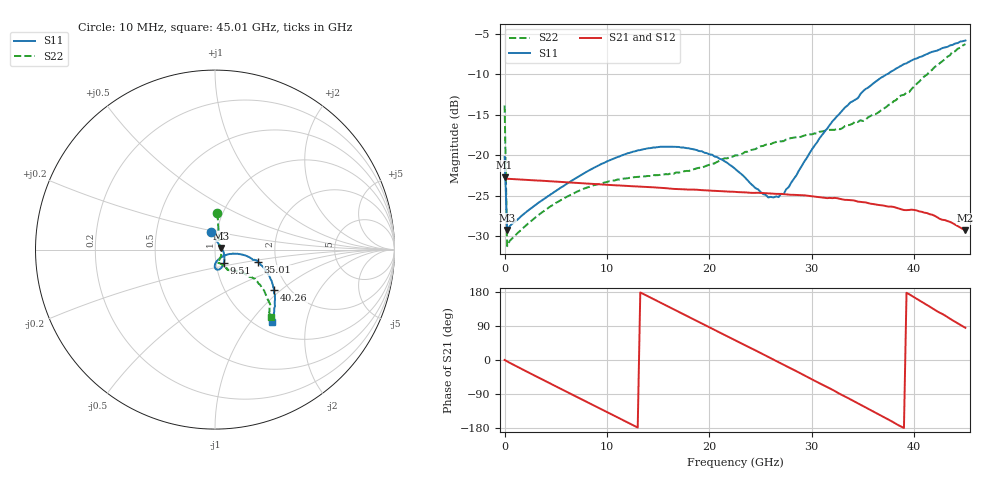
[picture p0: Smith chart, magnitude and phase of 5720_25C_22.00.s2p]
! Device:  ADRF5720
! Description: 0.5dB LSB GaAs MMIC 6-bit Digital Attenuator
! Frequency:  0.000009 -  40 GHz
! Ports:
!	RF1	= Port 1
!	RF2	= Port 2
! Vdd:  3.3 Volt
! Vss:  -3.3 Volt
! Control:  0/3.3 Volt
! State:  22.00 dB attenuation
! Data:  The device was measured using G-S-G Probes on a matrix board.
!  Data was collected using an calibrated 4 port network analyzer.
!  The reference plane for this measurement is at the launchers.
! Note:  Analog Devices supplies this data as a sample of measured data
!  for this product.  Your particular data for this product may vary.
!  Data was taken at 25 degrees C.
!  Analog Devices reserves the right to change this data at anytime.
# GHZ S DB R 45.0
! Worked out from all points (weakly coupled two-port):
!   181 points, 10 MHz to 45.01 GHz, reference 45 ohm
!   highest |S21| = -22.68 dB at 10 MHz (marker M1); lowest = -29.3 dB at 45.01 GHz (marker M2)
!   lowest |S11| = -29.2 dB at 260 MHz (marker M3), VSWR 1.07, Z = 48.1 + j0.87 ohm
!   |S11| at or under -10 dB: start of sweep to 37.31 GHz
!   |S22| runs from -31.2 to -6.2 dB; largest |S21 - S12| = 0.00011
!   S11 on the Smith chart (normalised r, x): 10 MHz: 0.94, +0.18; 9.51 GHz: 1.09, -0.16; 35.01 GHz: 1.61, -0.23; 40.26 GHz: 1.67, -0.89; 45.01 GHz: 1.16, -1.28
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0.01  -20.19 102.0  -22.68 0.0  -22.68 0.0  -13.83 86.2
0.26  -29.19 15.1  -22.88 -3.9  -22.88 -3.9  -31.20 16.9
0.51  -28.73 8.0  -22.89 -7.4  -22.90 -7.4  -30.54 6.9
3.26  -25.89 -17.8  -23.09 -45.5  -23.09 -45.5  -27.40 -34.0
7.76  -22.20 -47.3  -23.44 -106.9  -23.44 -106.9  -24.10 -67.0
9.51  -21.02 -55.9  -23.58 -130.6  -23.58 -130.6  -23.42 -73.2
12.51  -19.55 -68.5  -23.80 -171.4  -23.80 -171.4  -22.70 -78.1
15.26  -18.92 -78.1  -23.99 150.8  -23.99 150.8  -22.38 -77.0
19.26  -19.48 -88.7  -24.28 96.5  -24.28 96.5  -21.54 -68.7
21.26  -20.52 -90.7  -24.42 69.2  -24.42 69.2  -20.47 -64.4
22.76  -21.92 -89.7  -24.52 48.9  -24.52 48.9  -19.99 -61.9
25.76  -25.18 -62.9  -24.68 8.0  -24.68 8.1  -18.59 -59.4
26.76  -25.14 -46.1  -24.74 -5.6  -24.74 -5.5  -18.22 -58.2
27.76  -23.90 -29.2  -24.84 -19.4  -24.84 -19.4  -17.94 -58.0
30.26  -18.82 -11.3  -25.07 -54.3  -25.08 -54.2  -17.27 -56.2
32.26  -15.45 -10.8  -25.24 -81.9  -25.25 -81.9  -16.83 -52.8
35.01  -12.08 -16.0  -25.77 -121.4  -25.77 -121.4  -15.75 -46.5
37.76  -9.63 -25.3  -26.31 -161.0  -26.31 -160.9  -13.63 -39.0
40.26  -8.02 -34.5  -26.79 161.3  -26.80 161.4  -11.15 -36.1
42.26  -7.04 -41.6  -27.63 128.4  -27.64 128.4  -8.90 -40.0
43.76  -6.35 -47.0  -28.36 104.7  -28.36 104.7  -7.14 -45.1
45.01  -5.80 -52.1  -29.26 85.0  -29.26 85.0  -6.25 -50.5
